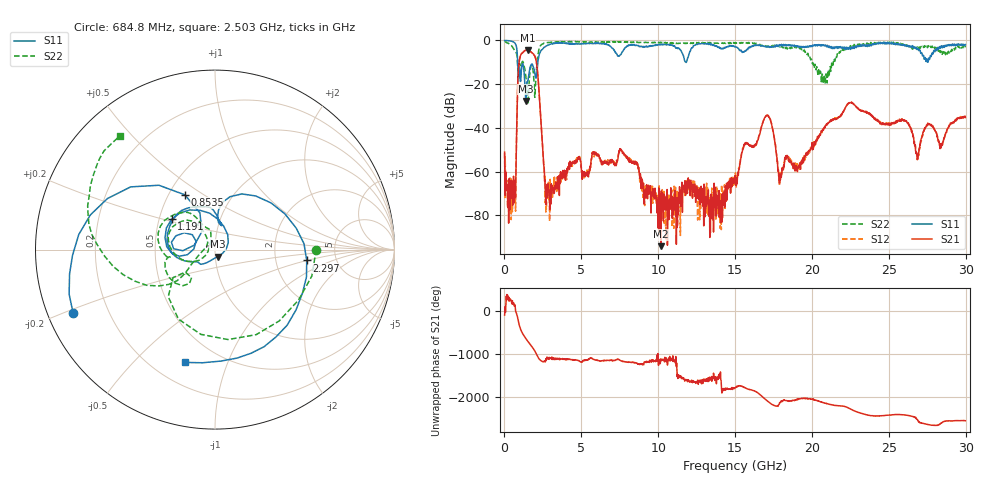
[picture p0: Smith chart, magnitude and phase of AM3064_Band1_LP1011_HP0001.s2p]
# Hz S DB R 50.0
!freq dBS11 angS11 dBS21 angS21 dBS12 angS12 dBS22 angS22
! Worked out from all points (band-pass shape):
!   1600 points, 10 MHz to 29.98 GHz, reference 50 ohm
!   highest |S21| = -4.39 dB at 1.51 GHz (marker M1); lowest = -94.0 dB at 10.17 GHz (marker M2)
!   |S21| within 3 dB of the highest: 1.023 GHz to 1.985 GHz (961.1 MHz wide, 63.9 % of centre)
!   lowest |S11| = -27.6 dB at 1.397 GHz (marker M3), VSWR 1.09, Z = 51.4 - j3.98 ohm
!   |S11| at or under -10 dB: 857.5 MHz to 2.171 GHz (1.313 GHz wide, 86.7 % of centre); 11.80225 GHz to 11.83018 GHz (27.92 MHz wide, 0.236 % of centre); 27.52553 GHz to 27.52764 GHz (2.111 MHz wide, 0.00767 % of centre)
!   |S22| runs from -29.1 to -0.3 dB; largest |S21 - S12| = 0.0074
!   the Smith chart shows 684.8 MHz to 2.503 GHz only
!   S11 on the Smith chart (normalised r, x): 684.8 MHz: 0.08, -0.21; 853.5 MHz: 0.60, +0.42; 1.191 GHz: 0.58, +0.22; 2.297 GHz: 3.03, -0.50; 2.503 GHz: 0.33, -0.72
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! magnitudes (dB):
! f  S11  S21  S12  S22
! 10 MHz  0.0  -51.1  -51.6  -0.3
! 366.1 MHz  -0.2  -77.4  -62.9  -1.8
! 684.8 MHz  -1.3  -71.2  -70.8  -5.0
! 853.5 MHz  -9.2  -22.2  -22.0  -11.0
! 1.191 GHz  -10.6  -5.6  -5.5  -9.6
! 1.397 GHz  -27.6  -4.4  -4.4  -17.0
! 1.51 GHz  -18.7  -4.4  -4.4  -25.7
! 2.297 GHz  -5.8  -28.6  -28.5  -2.9
! 2.503 GHz  -3.7  -50.6  -50.8  -1.7
! 2.803 GHz  -2.2  -69.3  -67.2  -1.0
! 5.015 GHz  -1.4  -60.3  -58.7  -0.7
! 7.639 GHz  -5.4  -50.3  -50.4  -0.7
! 10 GHz  -2.0  -81.9  -72.7  -1.0
! 10.17 GHz  -1.8  -94.0  -74.6  -0.9
! 15 GHz  -2.8  -61.7  -63.9  -1.4
! 17.05 GHz  -2.8  -34.3  -34.2  -2.8
! 17.93 GHz  -2.0  -61.0  -61.8  -2.4
! 19.99 GHz  -2.8  -49.0  -49.4  -9.4
! 22.45 GHz  -3.1  -28.5  -28.5  -3.5
! 25 GHz  -1.0  -38.3  -37.8  -1.0
! 26.87 GHz  -4.0  -54.1  -52.9  -3.1
! 29.98 GHz  -1.9  -35.3  -35.1  -3.2
